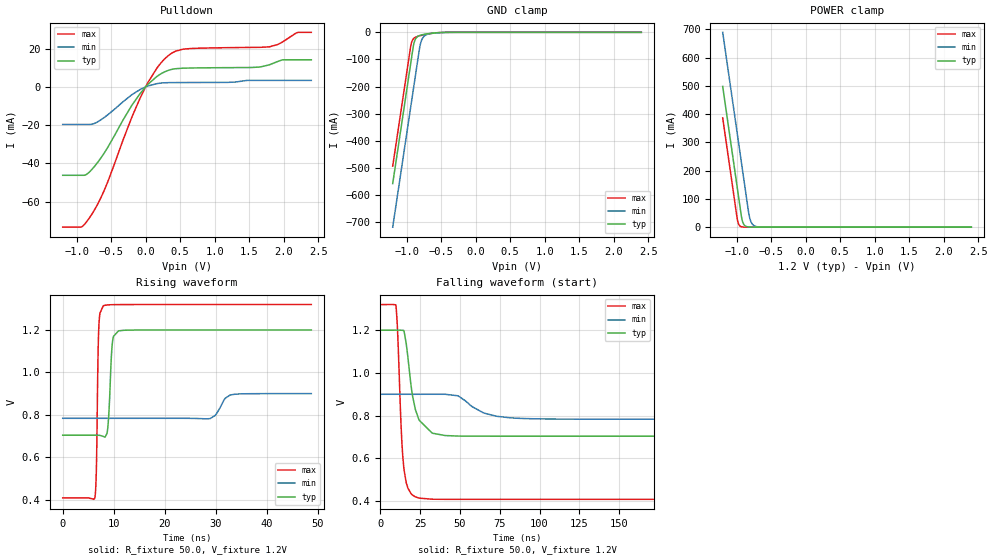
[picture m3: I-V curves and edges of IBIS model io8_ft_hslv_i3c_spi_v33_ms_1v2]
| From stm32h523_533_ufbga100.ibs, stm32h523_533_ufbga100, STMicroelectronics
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[Model]   io8_ft_hslv_i3c_spi_v33_ms_1v2
Model_type I/O_open_drain
Polarity   Non-Inverting
Enable   Active-Low
| CAP_THRESHOLD on pad IOFT is "UDTCAPC" :
| Rising=20.0% of vddiom   Falling=80.0% of vddiom
| C_comp min and max val. don't necessarily correlate with the min and max pvt
| but are the smallest and greatest pad capacitance found.
| var   typ   min   max
C_comp   3.39575pF  3.37230pF  3.42685pF
|C_comp_pulldown   3.39575pF  3.37230pF  3.42685pF
Vinl = 450.0mV
Vinh = 660.0mV
Vmeas = 600.0mV   | Reference voltage for timing measurements
Cref  = 50.0pF   | Timing specification test load capacitance value
Rref  = 1.0MOhm   | Timing specification test load resistance value
Vref  = 660.0mV   | Timing specification test load voltage
[Model Spec]
| TIME_THRESHOLD on pin ZII2CV11 is "CMOS" :
| Rising=40.0% of vdd   Falling=60.0% of vdd
Vinl 437.80000mV 335.80000mV 479.80000mV
Vinh 728.20000mV 529.20000mV 807.20000mV
| variable   typ   min   max
[Temperature Range] 25.0 125.0 -40.0
| variable   typ   min   max
[Voltage Range] 1.2V 900.0mV 1.32V
| variable   typ   min   max
[POWER Clamp Reference] 1.2V 900.0mV 1.32V
| variable   typ   min   max
[GND Clamp Reference] 0V 0V 0V
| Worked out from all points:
|   slope of the pulldown table from 0 to 0.18 V, typ, clamps not added: 30.6 ohm
|   GND clamp passes 1 mA (typ) near -0.52 V on its own axis
|   POWER clamp passes 1 mA (typ) near -0.84 V on its own axis
|   rising waveform, R_fixture 50.0, V_fixture 1.2V: 20-80 % time 571ps typ, 1.63ns min, 336ps max; typ from 0.704 V to 1.2 V
|   falling waveform, R_fixture 50.0, V_fixture 1.2V: 20-80 % time 6.35ns typ, 15.9ns min, 3.18ns max; typ from 1.2 V to 0.704 V
[POWER Clamp]
-1.2V     497.8mA    689.2mA    386.5mA
-990mV    140.8mA    332.2mA    29.53mA
-980mV    123.8mA    315.2mA    17.95mA
-960mV    89.81mA    281.2mA    6.634mA
-930mV    38.81mA    230.2mA    1.49mA
-900mV    12.07mA    179.2mA    334.8uA
-870mV    3.756mA    128.2mA    75.22uA
-820mV    536.4uA    44.98mA    6.246uA
-790mV    166.9uA    18.76mA    1.403uA
-750mV    35.18uA    5.846mA    191.8nA
-590mV    70.08nA    55uA       163.4pA
2.4V      0A         0A         0A
[GND Clamp]
-1.2V     -558.2mA   -719mA     -494.1mA
-940mV    -116.2mA   -277mA     -52.06mA
-930mV    -99.19mA   -260mA     -39.94mA
-900mV    -49.1mA    -209mA     -23.76mA
-880mV    -30.14mA   -175mA     -19.6mA
-850mV    -17.82mA   -124mA     -16.09mA
-810mV    -11.73mA   -56.78mA   -12.91mA
-780mV    -9.444mA   -28.21mA   -10.92mA
-740mV    -7.291mA   -13.16mA   -8.574mA
-640mV    -3.573mA   -4.171mA   -3.954mA
-380mV    -61.75uA   -230.3uA   -20.32uA
2.4V      3.863nA    718.6nA    150.6pA
| variable   typ   min   max
[Pullup Reference] 1.2V 900.0mV 1.32V
| variable   typ   min   max
[Pulldown Reference] 0V 0V 0V
[Pulldown]
-1.2V     -46.17mA   -19.62mA   -73.27mA
-930mV    -46.17mA   -19.62mA   -73.18mA
-770mV    -42.8mA    -19.41mA   -66.04mA
-570mV    -32.88mA   -15.18mA   -51.58mA
-80mV     -3.488mA   -1.363mA   -5.887mA
160mV     5.368mA    1.686mA    9.621mA
340mV     8.782mA    2.251mA    16.66mA
540mV     9.805mA    2.305mA    19.74mA
1.79V     11.53mA    3.428mA    20.94mA
1.98V     14.11mA    3.428mA    23.43mA
2.2V      14.2mA     3.428mA    28.44mA
2.4V      14.2mA     3.428mA    28.54mA
[Ramp]
dV/dt_r 297.78732mV/568.61782ps 69.82548mV/1.61345ns 547.12634mV/333.2193ps
dV/dt_f 297.80515mV/6.15704ns 69.92045mV/15.00298ns 547.13932mV/3.15799ns
R_load = 50.0
| Removed startup time: 0s 0s 0s  .
| Removed end time: 48.75ns.
[Rising Waveform]
R_fixture   = 50.0
V_fixture   = 1.2V
V_fixture_min = 900.0mV
V_fixture_max = 1.32V
0s        703.7mV    783.5mV    408.1mV
6.3ns     703.8mV    783.5mV    408.9mV
6.6ns     703.8mV    783.5mV    539.8mV
6.9ns     703.7mV    783.5mV    1.044V
7.05ns    703.5mV    783.5mV    1.195V
7.95ns    698mV      783.5mV    1.314V
8.85ns    741.4mV    783.5mV    1.318V
9.8ns     1.151V     783.5mV    1.319V
10.95ns   1.196V     783.5mV    1.32V
48.75ns   1.2V       899.8mV    1.32V
| Removed startup time: 0s 0s 0s  .
| Removed end time: 398.75ns.
[Falling Waveform]
R_fixture   = 50.0
V_fixture   = 1.2V
V_fixture_min = 900.0mV
V_fixture_max = 1.32V
0s        1.2V       900mV      1.32V
9.8ns     1.2V       900mV      1.318V
10.9ns    1.2V       900mV      1.189V
13.25ns   1.2V       900mV      721.5mV
14.9ns    1.196V     900mV      548.7mV
20.25ns   892.7mV    900mV      428mV
24.4ns    778.6mV    900mV      413.8mV
40.7ns    706.8mV    900mV      408.1mV
89.55ns   703.7mV    786.6mV    408.1mV
398.8ns   703.7mV    783.5mV    408.1mV
